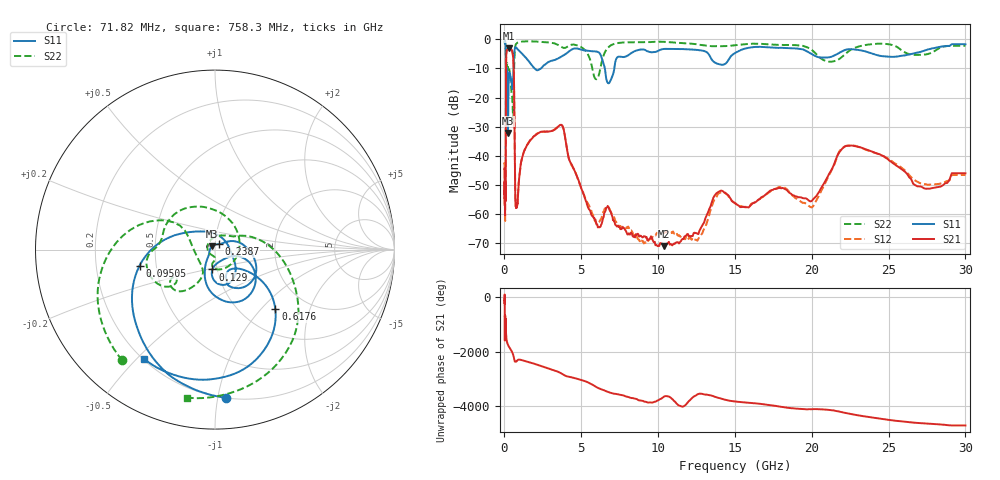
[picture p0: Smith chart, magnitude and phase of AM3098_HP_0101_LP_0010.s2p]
! Date/Time: Thu, Feb 28, 2019 8:36 AM
! Network Analyzer: Agilent Technologies E8364B Rev: A.07.50.67
! Sweep from 0.010 to 30.000 GHz, 1601 Points, Sweep Type: LOG
! Power Supply: 5.022 V, 0.002 A
# Hz S DB R 50
!freq MagS11 AngS11 MagS21 AngS21 MagS12 AngS12 MagS22 AngS22
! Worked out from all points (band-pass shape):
!   1601 points, 10 MHz to 30 GHz, reference 50 ohm
!   highest |S21| = -3.03 dB at 266.5 MHz (marker M1); lowest = -71.2 dB at 10.38 GHz (marker M2)
!   |S21| within 3 dB of the highest: 113.4 MHz to 562.9 MHz (449.5 MHz wide, 133 % of centre)
!   lowest |S11| = -32.2 dB at 230.5 MHz (marker M3), VSWR 1.05, Z = 48.5 + j1.87 ohm
!   |S11| at or under -10 dB: 176 MHz to 588 MHz (412 MHz wide, 108 % of centre); 1.966 GHz to 2.381 GHz (414.3 MHz wide, 19.1 % of centre); 6.531 GHz to 7.148 GHz (616.4 MHz wide, 9.01 % of centre)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
!   |S22| runs from -29.0 to -0.5 dB; largest |S21 - S12| = 0.013
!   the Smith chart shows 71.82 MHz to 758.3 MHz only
!   S11 on the Smith chart (normalised r, x): 71.82 MHz: 0.20, -1.05; 95.05 MHz: 0.40, -0.09; 129 MHz: 0.95, -0.21; 238.7 MHz: 1.04, +0.06; 617.6 MHz: 1.41, -1.21; 758.3 MHz: 0.20, -0.52
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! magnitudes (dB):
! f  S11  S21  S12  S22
! 10 MHz  -0.4  -44.8  -43.0  -0.5
! 38.04 MHz  -0.5  -59.1  -60.9  -0.8
! 71.82 MHz  -1.6  -53.4  -53.0  -1.9
! 80.98 MHz  -2.4  -52.6  -49.5  -2.7
! 95.05 MHz  -7.3  -22.6  -22.4  -8.6
! 129 MHz  -19.0  -4.5  -4.5  -10.6
! 144.7 MHz  -16.7  -3.8  -3.8  -10.9
! 186.8 MHz  -11.2  -3.5  -3.5  -8.2
! 230.5 MHz  -32.2  -3.1  -3.1  -9.9
! 238.7 MHz  -28.5  -3.1  -3.1  -10.0
! 266.5 MHz  -15.5  -3.0  -3.0  -10.4
! 550.5 MHz  -15.0  -5.4  -5.4  -25.1
! 617.6 MHz  -6.5  -13.4  -13.3  -13.2
! 758.3 MHz  -2.8  -57.8  -57.9  -1.5
! 2.084 GHz  -10.5  -32.7  -32.5  -0.7
! 3.723 GHz  -5.8  -29.5  -29.5  -2.6
! 5.989 GHz  -4.2  -63.5  -63.7  -13.7
! 7.926 GHz  -5.8  -66.2  -64.8  -1.0
! 10.38 GHz  -3.3  -71.2  -66.6  -0.8
! 19.8 GHz  -4.5  -55.5  -57.3  -3.0
! 22.67 GHz  -3.4  -36.6  -36.5  -3.2
! 30 GHz  -1.6  -46.1  -46.7  -2.2
